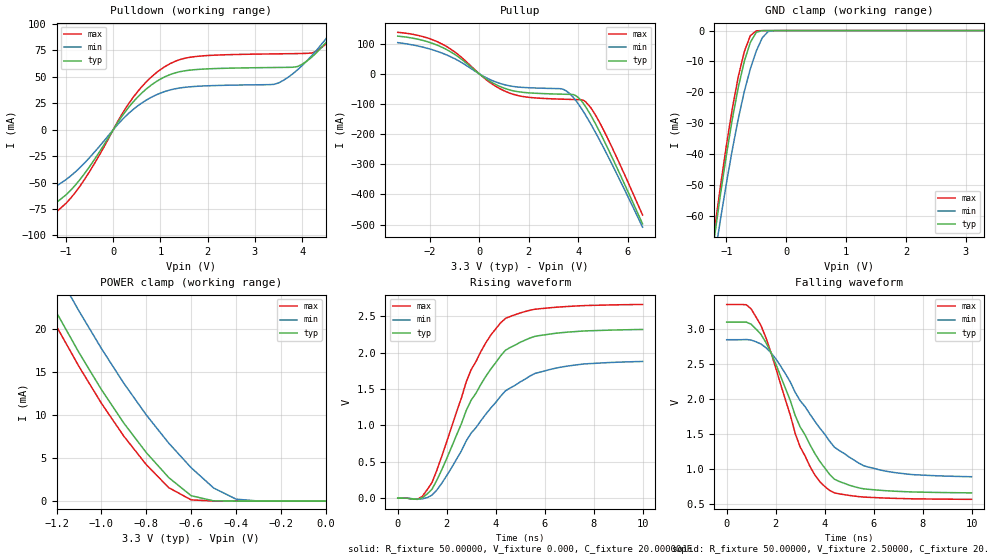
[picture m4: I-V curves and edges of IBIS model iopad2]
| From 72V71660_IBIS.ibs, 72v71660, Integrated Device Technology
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|   Model iopad2
[Model]   iopad2
Model_type   3-state
Polarity   Non-Inverting
Enable   Active-High
|Vinl =  0.80000V
|Vinh =  2.00000V
Vmeas =  1.50000V
C_comp   5.00000pF   NA   NA
[Temperature Range]   25.00000   100.00000   0.000
[Voltage Range]   3.30000V   3.00000V   3.60000V
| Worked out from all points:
|   slope of the pulldown table from 0 to 0.495 V, typ, clamps not added: 16.6 ohm
|   slope of the pullup table from 0 to 0.495 V, typ, clamps not added: 17.8 ohm
|   GND clamp passes 1 mA (typ) near -0.51 V on its own axis
|   POWER clamp passes 1 mA (typ) near -0.62 V on its own axis
|   rising waveform, R_fixture 50.00000, V_fixture 0.000, C_fixture 20.00000pF: 20-80 % time 2.09ns typ, 2.42ns min, 1.83ns max; typ from 0 V to 2.32 V
|   falling waveform, R_fixture 50.00000, V_fixture 2.50000, C_fixture 20.00000pF: 20-80 % time 1.86ns typ, 2.3ns min, 1.6ns max; typ from 3.1 V to 0.664 V
[Pulldown]
| voltage   I(typ)   I(min)   I(max)
-3.3V     -98.4mA    -81.6mA    -110.5mA
-1.9V     -86.7mA    -69mA      -97.4mA
-1.3V     -72.39mA   -56.23mA   -81.62mA
-700mV    -46.93mA   -35.66mA   -53.13mA
500mV     30.13mA    21.95mA    35.15mA
1.3V      53.65mA    38.64mA    64.55mA
3.5V      58.92mA    44.27mA    71.82mA
4V        61.98mA    60.77mA    72.15mA
4.3V      72.72mA    74.98mA    74.19mA
4.7V      93.71mA    97.88mA    90.11mA
4.9V      106.9mA    111.1mA    101.7mA
6.6V      332.3mA    305.7mA    332.7mA
[Pullup]
| voltage   I(typ)   I(min)   I(max)
-3.3V     125.2mA    103.6mA    137.8mA
-2.3V     111.4mA    89.05mA    124mA
-1.5V     87.92mA    68.7mA     98.72mA
400mV     -23.22mA   -17.71mA   -26.92mA
1.2V      -52.71mA   -39.4mA    -62.98mA
3.3V      -67.33mA   -49.39mA   -83.88mA
3.6V      -67.91mA   -61.92mA   -84.61mA
4V        -78.45mA   -99.51mA   -85.44mA
4.2V      -97.4mA    -124.1mA   -87.42mA
4.5V      -136.2mA   -165.3mA   -111.4mA
5.3V      -265.2mA   -289.4mA   -232.6mA
6.6V      -497.9mA   -508.6mA   -468.4mA
[GND_clamp]
| voltage   I(typ)   I(min)   I(max)
-3.3V     -424.5mA   -403.9mA   -432.6mA
-1.2V     -66.92mA   -73.75mA   -64.72mA
-1.1V     -53.15mA   -61.24mA   -50.45mA
-900mV    -28.53mA   -38.43mA   -25.1mA
-800mV    -18.24mA   -28.42mA   -14.77mA
-700mV    -9.881mA   -19.65mA   -6.763mA
-600mV    -3.825mA   -12.36mA   -1.625mA
-500mV    -527.4uA   -6.58mA    -76.57uA
-400mV    -20.22uA   -2.288mA   -6.836uA
-300mV    -3.602uA   -280.8uA   -3.979uA
-200mV    -2.123uA   -15.65uA   -2.592uA
3.3V      10.56uA    18.9uA     14.69uA
[POWER_clamp]
| voltage   I(typ)   I(min)   I(max)
-3.3V     169.2mA    163.5mA    171.9mA
-1.3V     26.9mA     31.61mA    25.33mA
-1.2V     21.94mA    26.75mA    20.33mA
-1.1V     17.29mA    22.12mA    15.67mA
-1V       12.98mA    17.76mA    11.39mA
-900mV    9.076mA    13.71mA    7.557mA
-800mV    5.648mA    10.03mA    4.252mA
-700mV    2.746mA    6.756mA    1.573mA
-600mV    637.5uA    3.891mA    149.6uA
-500mV    36.76uA    1.536mA    17.14uA
-400mV    11.14uA    236.2uA    14.74uA
0V        10.56uA    6.266uA    14.69uA
[Ramp]
| variable   typ   min   max
dV/dt_r   1.39320/1.55930n   1.13040/1.91193n   1.59900/1.33876n
dV/dt_f   1.40082/1.59343n   1.10280/2.00920n   1.61130/1.37344n
R_load = 50.00000
[Rising Waveform]
R_fixture = 50.00000
V_fixture = 0.000
C_fixture = 20.00000pF
R_dut = 129.80000m
L_dut = 9.76000nH
C_dut = 1.23400pF
| time   V(typ)   V(min)   V(max)
0s        0V         0V         0V
800ps     -15.34mV   -14.73mV   -14.68mV
1.4ns     123.2mV    42.12mV    215.7mV
2ns       544.3mV    309.9mV    775.3mV
3ns       1.346V     894.2mV    1.765V
3.8ns     1.772V     1.238V     2.238V
4.4ns     2.031V     1.474V     2.468V
5.6ns     2.221V     1.712V     2.594V
6.4ns     2.262V     1.781V     2.619V
10ns      2.316V     1.877V     2.659V
[Falling Waveform]
R_fixture = 50.00000
V_fixture = 2.50000
C_fixture = 20.00000pF
R_dut = 129.80000m
L_dut = 9.76000nH
C_dut = 1.23400pF
| time   V(typ)   V(min)   V(max)
0s        3.103V     2.852V     3.355V
800ps     3.104V     2.855V     3.352V
1.4ns     2.929V     2.791V     3.055V
2ns       2.51V      2.582V     2.453V
3ns       1.606V     1.981V     1.32V
3.6ns     1.226V     1.687V     920.1mV
4.2ns     929.7mV    1.404V     700mV
4.6ns     825.6mV    1.268V     648.8mV
5.8ns     713.7mV    1.031V     599.6mV
10ns      663.6mV    894.1mV    570.9mV
